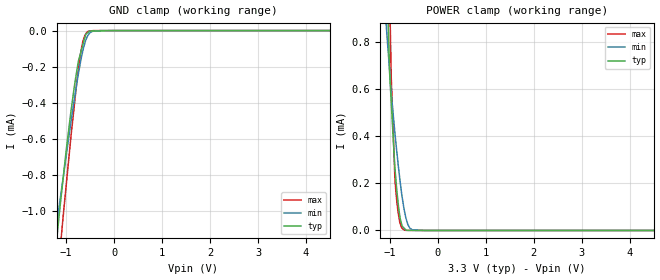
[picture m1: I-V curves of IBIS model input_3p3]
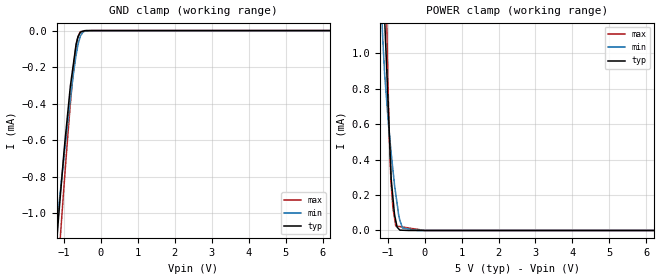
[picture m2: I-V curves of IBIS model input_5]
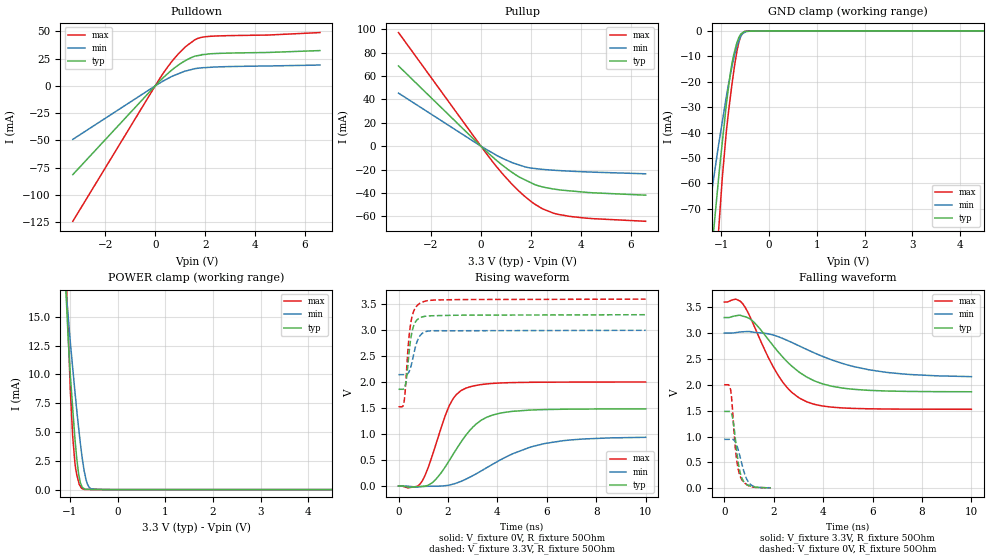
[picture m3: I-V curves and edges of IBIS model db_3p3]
|Texas Instruments Incorporated
| 12-bit, Dual Channel, Parallel Input, Multiplying Digital-to-Analog Converter
| Marketing part#   Digital Voltage Range   Package-type   #pins
| DAC7822IRTAR   2.5V - 5.5V   WQFN   40
| DAC7822IRTARG4   2.5V - 5.5V   WQFN   40
| DAC7822IRTAT   2.5V - 5.5V   WQFN   40
| DAC7822IRTATG4   2.5V - 5.5V   WQFN   40
[IBIS Ver]   3.2
[File name]   dac7822.ibs
|SIMDE Ver   V3.0 - 201101 - RHL4 - Build 457
[File Rev]   1.0
[Date]   6/20/2011
[Source]
| Texas Instruments Incorporated.
| Analog-eLab Design Center, HPA
| 12500 TI Blvd
| Dallas, TX -75243
| e-mail: elab_scm_ibis@list.ti.com
[Notes]   Revision History:
| Rev 1.0: 6/20/2011
| - Initial version of the model
| - Model generated from simulations in TISPICE
| - Model matched to SPICE simulation
| - C_comp although listed in numerical order of value are
|   obtained from varying PVT conditions. For PVT conditions for
|   each specific value refer the buffer description under
|   respective [Model]. IBIS model user is responsible for using
|   appropriate C_comp to simulate for Signal Integrity.
| - Model names with a trailing _3p3 contains the model for
|   3.3V [3.0V and 3.6V]. Model names with a trailing _5 contains
|   the model for 5.0V [4.5V and 5.5V].
[Disclaimer]
| This model is designed as an aid for customers of Texas Instruments.
| TI and its licensors and suppliers make no warranties, either expressed
| or implied, with respect to this  model, including the warranties of
| merchantability or fitness for a particular purpose. The model is
| provided solely on an "as is" basis. The entire risk as to its quality
| and performance is with the customer.
[Copyright]
 (C) Copyright 2011 Texas Instruments Incorporated.All rights reserved.
|   DAC7822
[Component]   DAC7822
[Manufacturer]   TI
[Package]   |40 WQFN   -  RTA package
|   typ   min   max
R_pkg   0.10977   0.09279   0.12930
L_pkg   1.92171nH   1.57794nH   2.31474nH
C_pkg   0.41350pF   0.38926pF   0.44761pF
[Pin]  signal_name   model_name   R_pin   L_pin   C_pin
1   R1A   TERM   0.12203   2.17064nH  0.43159pF
2   R2A   TERM   0.10523   1.83674nH  0.41098pF
3   R2_3A   TERM   0.09781   1.69014nH  0.40320pF
4   R3A   TERM   0.09347   1.60464nH  0.39540pF
5   VREFA   TERM   0.09279   1.59134nH  0.38926pF
6   DGND   GND   0.09441   1.62324nH  0.39108pF
7   _LDAC   INPUT   0.09894   1.71244nH  0.40089pF
8   DAC_A/B   INPUT   0.10588   1.84964nH  0.40646pF
9   NC   NC   0.00015   0.00114nH  0.26369pF
10   DB11   DB   0.12930   2.31474nH  0.43408pF
11   DB10   DB   0.12519   2.23134nH  0.42874pF
12   DB9   DB   0.11079   1.94464nH  0.40955pF
13   DB8   DB   0.10554   1.83974nH  0.40813pF
14   DB7   DB   0.10055   1.73964nH  0.40024pF
15   DB6   DB   0.09877   1.70344nH  0.39465pF
16   DB5   DB   0.09877   1.70234nH  0.39477pF
17   DB4   DB   0.10055   1.73664nH  0.40008pF
18   DB3   DB   0.10554   1.83434nH  0.40747pF
19   DB2   DB   0.11079   1.93774nH  0.40956pF
20   DB1   DB   0.12519   2.22404nH  0.42902pF
21   DB0   DB   0.12930   2.30474nH  0.44761pF
22   _CS   INPUT   0.11937   2.10634nH  0.43858pF
23   R/_W   INPUT   0.10973   1.91434nH  0.41989pF
24   _CLR   INPUT   0.10184   1.75734nH  0.40694pF
25   VDD   POWER   0.09613   1.64414nH  0.39802pF
26   VREFB   TERM   0.09279   1.57794nH  0.39379pF
27   R3B   TERM   0.00015   0.00114nH  0.26320pF
28   R2_3B   TERM   0.00015   0.00114nH  0.26378pF
29   R2B   TERM   0.00015   0.00114nH  0.26362pF
30   R1B   TERM   0.12203   2.15884nH  0.43153pF
31   RFBB   TERM   0.12535   2.22624nH  0.43928pF
32   IOUT2B   GND   0.11704   2.06124nH  0.42682pF
33   IOUT1B   TERM   0.11028   1.92764nH  0.40343pF
34   NC   NC   0.00015   0.00114nH  0.26358pF
35   NC   NC   0.00015   0.00114nH  0.26344pF
36   NC   NC   0.00015   0.00114nH  0.26352pF
37   NC   NC   0.00015   0.00114nH  0.26376pF
38   IOUT1A   TERM   0.11028   1.93454nH  0.40340pF
39   IOUT2A   GND   0.11704   2.06954nH  0.42697pF
40   RFBA   TERM   0.12535   2.23574nH  0.43956pF
41   THERMAL_PAD   NC   0.00015   0.00114nH  4.29466pF
|   Model Selectors
[Model Selector] INPUT
input_3p3   3.3V digital input
input_5   5.0V digital input
[Model Selector] DB
db_3p3   3.3V digital i/o
db_5   5.0V digital i/o
[Model Selector] TERM
term_3-3V  3.3V nominal termination
term_5-0V  5.0V nominal termination
[Model] term_3-3V
Model_type Terminator
C_comp   1.0e-20F  1.0e-20F  1.0e-20F
|   typ   min   max
[Voltage Range]   3.3V   3.0V   3.6V
[POWER Clamp Reference]   3.3V   3.0V   3.6V
[GND Clamp Reference]   0V   0V   0V
|Ambient Temperature   25   125   -40
|Junction Temperature
[Temperature Range]   25   125   -40
[Model] term_5-0V
Model_type Terminator
C_comp   1.0e-20F  1.0e-20F  1.0e-20F
|   typ   min   max
[Voltage Range]   5.0V   4.5V   5.5V
[POWER Clamp Reference]   5.0V   4.5V   5.5V
[GND Clamp Reference]   0V   0V   0V
|Ambient Temperature   25   125   -40
|Junction Temperature
[Temperature Range]   25   125   -40
| Models and submodels in the file (6): input_3p3 (Input), input_5 (Input), db_3p3 (I/O), db_5 (I/O), term_3-3V (Terminator), term_5-0V (Terminator)
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|   input_3p3 Model
[Model]   input_3p3
Model_type   Input
Vinl = 0.6
Vinh = 2.1
|   typ   min   max
|   (nom PVT)   (fast PVT)   (slow PVT)
|C_comp from frequency sweep method (F=66.67MHz)
|Average
|C_comp   4.767e-13   4.760e-13   4.773e-13
|C_comp from LC tank measurement(L=1nH)
|Average
|Resonant Frequency(Hz)   8.760e+09   8.930e+09   8.530e+09
C_comp   3.304e-13   3.180e-13   3.485e-13
| Where nom  PVT is Nominal Process, 3.3V, 25C
|   Fast PVT is Strong Process,  3.6V, -40C
|   Slow PVT is Weak Process,   3V, 125C
[Voltage Range]   3.3   3   3.6
|Ambient Temperature   25   125   -40
|Junction Temperature
[Temperature Range]   25   125   -40
[Power Clamp Reference]   3.3   3   3.6
[GND Clamp Reference]   0   0   0
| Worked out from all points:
|   GND clamp passes 1 mA (typ) near -1.14 V on its own axis
|   POWER clamp passes 1 mA (typ) near -1.05 V on its own axis
[GND Clamp]
|   Voltage   I(typ)   I(min)   I(max)
-3.3V     -6.935mA   -5.364mA   -9.228mA
-1.213V   -1.199mA   -1.108mA   -1.47mA
-1.149V   -1.033mA   -980.4uA   -1.282mA
-1.112V   -938.6uA   -910.1uA   -1.174mA
-1.066V   -826.3uA   -821.6uA   -1.038mA
-897.6mV  -443.2uA   -501.8uA   -581.9uA
-730.8mV  -156.3uA   -219.4uA   -187uA
-648mV    -75.46uA   -107.1uA   -58.31uA
-590.7mV  -19.5uA    -52.96uA   -18.66uA
-532.8mV  -7.468uA   -21.95uA   -3.584uA
-285mV    -1.686uA   -83.41nA   -82.96nA
6.6V      0A         0A         0A
[POWER Clamp]
|   Voltage   I(typ)   I(min)   I(max)
-3.3V     29.6mA     22.19mA    37.43mA
-1.089V   1.261mA    909.4uA    2.005mA
-1.051V   997.3uA    804.4uA    1.493mA
-1.003V   661.9uA    671uA      984.4uA
-896.4mV  270.2uA    418.1uA    227.3uA
-874.8mV  217.3uA    374.1uA    166uA
-792mV    59.64uA    217.2uA    34.48uA
-745.8mV  19.16uA    144.6uA    10.15uA
-702mV    9.822uA    88.04uA    2.044uA
-624mV    517.4nA    24.99uA    505.2nA
-534mV    442.4nA    2.793uA    259.2nA
6.6V      0A         0A         0A
|   input_5 Model
[Model]   input_5
Model_type   Input
Vinl = 0.8
Vinh = 2.4
|   typ   min   max
|   (nom PVT)   (fast PVT)   (slow PVT)
|C_comp from frequency sweep method (F=66.67MHz)
|Average
|C_comp   4.622e-13   4.612e-13   4.629e-13
|C_comp from LC tank measurement(L=1nH)
|Average
|Resonant Frequency(Hz)   8.760e+09   8.930e+09   8.530e+09
C_comp   3.304e-13   3.180e-13   3.485e-13
| Where nom  PVT is Nominal Process, 5V, 25C
|   Fast PVT is Strong Process,  5.5V, -40C
|   Slow PVT is Weak Process,   4.5V, 125C
[Voltage Range]   5   4.5   5.5
|Ambient Temperature   25   125   -40
|Junction Temperature
[Temperature Range]   25   125   -40
[Power Clamp Reference]   5   4.5   5.5
[GND Clamp Reference]   0   0   0
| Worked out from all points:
|   GND clamp passes 1 mA (typ) near -1.14 V on its own axis
|   POWER clamp passes 1 mA (typ) near -1.04 V on its own axis
[GND Clamp]
|   Voltage   I(typ)   I(min)   I(max)
-5V       -11.54mA   -8.806mA   -15.47mA
-1.26V    -1.322mA   -1.2mA     -1.615mA
-1.139V   -1.005mA   -959.8uA   -1.247mA
-994.5mV  -655.3uA   -682.2uA   -841.2uA
-825mV    -303uA     -374.6uA   -398.4uA
-748mV    -189.2uA   -245.2uA   -222.2uA
-682mV    -91.77uA   -149.2uA   -101.4uA
-632.5mV  -44.34uA   -92.24uA   -43.64uA
-550mV    -7.983uA   -28.52uA   -5.917uA
-481.5mV  -3.441uA   -7.411uA   -3.301uA
-261mV    -214.4nA   -46.74nA   -23.29nA
10V       0A         0A         0A
[POWER Clamp]
|   Voltage   I(typ)   I(min)   I(max)
-5V       52.24mA    40.05mA    65.2mA
-1.144V   1.78mA     1.135mA    2.733mA
-1.08V    1.185mA    878.5uA    1.86mA
-1.067V   1.119mA    842.9uA    1.691mA
-1.006V   810.6uA    677.1uA    980.6uA
-957mV    558.3uA    551.7uA    536.6uA
-905mV    293.3uA    436.6uA    259.6uA
-858mV    185.9uA    342.8uA    128.6uA
-781mV    55.37uA    205.7uA    25.62uA
-670mV    1.936uA    56.56uA    21.98uA
-202.5mV  0A         0A         6.644uA
10V       0A         0A         0A
|   db_3p3 Model
[Model]   db_3p3
Model_type   I/O
Polarity   Non-Inverting
Enable   Active-Low
Vinl = 0.6
Vinh = 2.1
Vmeas = 1.65
Vref = 1.65
Cref = 2pF
Rref = 50
|   typ   min   max
|   (nom PVT)   (fast PVT)   (slow PVT)
|C_comp from frequency sweep method (F=83.3MHz)
C_comp   2.771e-12   2.729e-12   3.034e-12
|ON state : BUFFER OUTPUT TURNED HIGH
|C_comp   4.377e-12   4.259e-12   4.424e-12
|OFF state: BUFFER IN HIGH IMPEDANCE
|C_comp   2.771e-12   2.729e-12   3.034e-12
|C_comp from LC tank measurement(L=1nH)
|Average
|Resonant Frequency(Hz)   3.235e+09   3.240e+09   3.120e+09
|C_comp   2.423e-12   2.415e-12   2.605e-12
|ON state : BUFFER OUTPUT TURNED HIGH
|Resonant Frequency(Hz)   3.220e+09   3.220e+09   3.100e+09
|C_comp   2.445e-12   2.445e-12   2.638e-12
|OFF state: BUFFER IN HIGH IMPEDANCE
|Resonant Frequency(Hz)   3.250e+09   3.260e+09   3.140e+09
|C_comp   2.401e-12   2.386e-12   2.572e-12
| Where nom  PVT is Nominal Process, 3.3V, 25C
|   Fast PVT is Strong Process,  3.6V, -40C
|   Slow PVT is Weak Process,   3V, 125C
[Voltage Range]   3.3   3   3.6
|Ambient Temperature   25   125   -40
|Junction Temperature
[Temperature Range]   25   125   -40
[Pullup Reference]   3.3   3   3.6
[Pulldown Reference]   0   0   0
[Power Clamp Reference]   3.3   3   3.6
[GND Clamp Reference]   0   0   0
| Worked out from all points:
|   slope of the pulldown table from 0 to 0.495 V, typ, clamps not added: 44.5 ohm
|   slope of the pullup table from 0 to 0.495 V, typ, clamps not added: 50.9 ohm
|   GND clamp passes 1 mA (typ) near -0.57 V on its own axis
|   POWER clamp passes 1 mA (typ) near -0.80 V on its own axis
|   falling waveform, V_fixture 3.3V, R_fixture 50Ohm: 20-80 % time 1.77ns typ, 2.82ns min, 1.39ns max; typ from 3.3 V to 1.87 V
|   rising waveform, V_fixture 0V, R_fixture 50Ohm: 20-80 % time 1.34ns typ, 2.39ns min, 883ps max; typ from 0 V to 1.49 V
|   rising waveform, V_fixture 3.3V, R_fixture 50Ohm: 20-80 % time 227ps typ, 283ps min, 225ps max; typ from 1.86 V to 3.3 V
|   falling waveform, V_fixture 0V, R_fixture 50Ohm: 20-80 % time 251ps typ, 335ps min, 227ps max; typ from 1.49 V to 0.01 V
[Pulldown]
|   Voltage   I(typ)   I(min)   I(max)
-3.3V     -81.5mA    -49.13mA   -124.4mA
172.8mV   4.174mA    2.439mA    6.404mA
684mV     14.89mA    8.867mA    22.88mA
939.6mV   19.32mA    11.24mA    29.68mA
1.246V    23.69mA    13.79mA    36.53mA
1.588V    27.25mA    15.81mA    42.3mA
1.829V    28.22mA    16.53mA    44.46mA
2.012V    28.87mA    16.82mA    45.15mA
2.627V    29.91mA    17.52mA    45.94mA
4.5V      30.68mA    18.26mA    46.67mA
6.6V      32.42mA    19.13mA    48.96mA
[GND Clamp]
|   Voltage   I(typ)   I(min)   I(max)
-3.3V     -572.6mA   -390.1mA   -824.3mA
-1.422V   -133mA     -93.55mA   -191.1mA
-1.267V   -99.78mA   -71.9mA    -141.4mA
-1.211V   -88.13mA   -64.44mA   -124.3mA
-1.098V   -65.74mA   -49.69mA   -89.8mA
-1.062V   -58.61mA   -45.19mA   -79.43mA
-1.04V    -54.15mA   -42.56mA   -73.38mA
-896.4mV  -28.9mA    -25.83mA   -39.52mA
-774mV    -12.45mA   -13.61mA   -20.35mA
-633.6mV  -2.577mA   -3.997mA   -4.428mA
-514.8mV  -213.6uA   -665uA     -263uA
6.6V      0A         0A         0A
[Pullup]
|   Voltage   I(typ)   I(min)   I(max)
-3.3V     68.69mA    45.42mA    97.3mA
40.16fV   0A         0A         -1.07fA
478.8mV   -9.421mA   -6.009mA   -13.57mA
939.6mV   -17.62mA   -11.14mA   -25.45mA
1.278V    -22.88mA   -14.35mA   -33.32mA
1.554V    -26.67mA   -16.25mA   -39.07mA
1.994V    -31.21mA   -18.74mA   -47.15mA
2.473V    -34.92mA   -19.89mA   -53.74mA
2.927V    -36.77mA   -20.62mA   -57.53mA
3.557V    -38.27mA   -21.39mA   -60.15mA
4.5V      -39.96mA   -22.26mA   -62.11mA
6.6V      -41.98mA   -23.67mA   -64.35mA
[POWER Clamp]
|   Voltage   I(typ)   I(min)   I(max)
-3.3V     231.5mA    181.1mA    292mA
-1.128V   20.91mA    19.56mA    23.96mA
-1.033V   12.73mA    14.81mA    13.18mA
-993.6mV  9.994mA    12.84mA    8.722mA
-943.2mV  7.076mA    10.58mA    4.625mA
-896.4mV  4.423mA    8.502mA    2.3mA
-818.4mV  1.35mA     5.35mA     657.8uA
-785.4mV  636.2uA    4.109mA    307.2uA
-702mV    87.39uA    1.615mA    15.83uA
-633mV    23.15uA    459.9uA    9.331uA
-552mV    20.17uA    58.14uA    5.431uA
6.6V      0A         0A         0A
[Ramp]
R_load = 50
|   typ   min   max
dV/dt_r   0.891748/1.3398e-09   0.563269/2.39143e-09   1.20247/8.77693e-10
dV/dt_f   0.860362/1.77097e-09   0.504996/2.80324e-09   1.24326/1.38847e-09
[Falling Waveform]
V_fixture = 3.3V
V_fixture_min = 3V
V_fixture_max = 3.6V
R_fixture = 50Ohm
|   Time   V(typ)   V(min)   V(max)
0s        3.3V       3V         3.6V
467ps     3.334V     3.01V      3.656V
742ps     3.329V     3.025V     3.572V
1.25ns    3.187V     3.012V     3.094V
2.229ns   2.611V     2.922V     2.149V
2.732ns   2.362V     2.819V     1.856V
3.308ns   2.159V     2.69V      1.679V
4.352ns   1.973V     2.481V     1.569V
5.88ns    1.893V     2.289V     1.537V
10ns      1.866V     2.158V     1.528V
[Rising Waveform]
V_fixture = 0V
V_fixture_min = 0V
V_fixture_max = 0V
R_fixture = 50Ohm
|   Time   V(typ)   V(min)   V(max)
0s        1.322nV    1.922nV    1.112nV
918ps     -7.24mV    -10.81mV   67.84mV
1.403ns   79.98mV    -3.205mV   639.7mV
2.062ns   497.9mV    20.26mV    1.556V
2.343ns   712.9mV    57.15mV    1.764V
2.721ns   976.1mV    131.2mV    1.884V
3.332ns   1.263V     287.9mV    1.954V
3.787ns   1.364V     414.5mV    1.976V
5.9ns     1.473V     817mV      2V
10ns      1.486V     938.8mV    2.004V
[Rising Waveform]
V_fixture = 3.3V
V_fixture_min = 3V
V_fixture_max = 3.6V
R_fixture = 50Ohm
|   Time   V(typ)   V(min)   V(max)
0s        1.864V     2.146V     1.527V
169ps     1.863V     2.146V     1.535V
231ps     1.879V     2.145V     1.641V
318ps     2.06V      2.147V     2.163V
413ps     2.499V     2.19V      2.81V
476ps     2.771V     2.264V     3.076V
542ps     2.96V      2.379V     3.254V
744ps     3.197V     2.773V     3.471V
953ps     3.257V     2.939V     3.542V
10ns      3.3V       2.999V     3.6V
[Falling Waveform]
V_fixture = 0V
V_fixture_min = 0V
V_fixture_max = 0V
R_fixture = 50Ohm
|   Time   V(typ)   V(min)   V(max)
0s        1.486V     947mV      2.001V
192ps     1.487V     946.9mV    1.995V
262ps     1.473V     948mV      1.895V
348ps     1.339V     944.7mV    1.435V
421ps     1.079V     918.2mV    939.2mV
487ps     799mV      859.4mV    611.8mV
654ps     285.8mV    586mV      224.2mV
870ps     88.78mV    223.4mV    86.21mV
1.055ns   44.95mV    78.08mV    36.12mV
1.884ns   10.22mV    9.301mV    11.42mV
